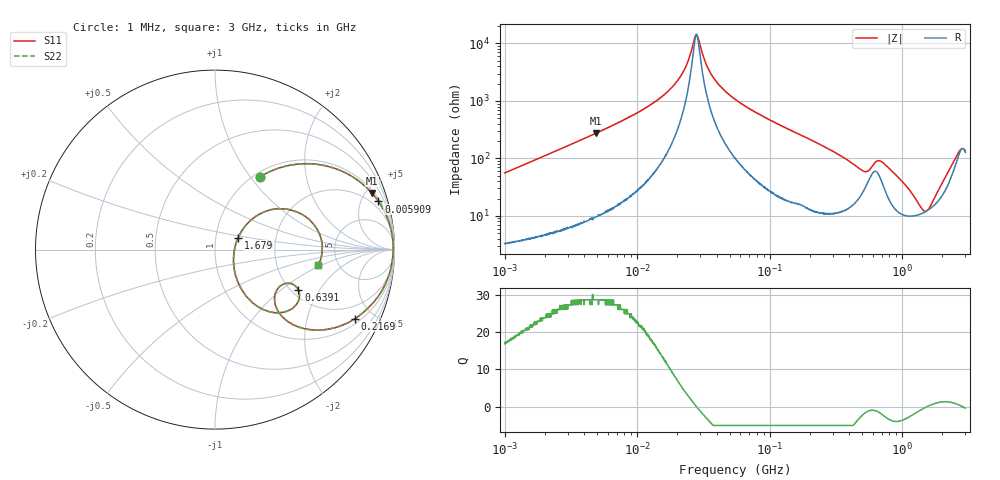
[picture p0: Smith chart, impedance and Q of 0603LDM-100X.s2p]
!s-Parameter Generated by FASTRON Sdn. Bhd.
!FASTRON P/N : 0603LDM-100X
!Keysight Technologies: E4991B_MY54100416_A.01.15
!Date: Thu Nov 27 16:25:48 2025
!Version  :Rev00  Thu Nov 27 16:25:48 2025
!Data & Calibration Information:
!Freq  S11  S21  S12  S22
!PortZ  Port1:50+j0  Port2:50+j0
!When reading reference impedance value at option line is always used.
! Remarks : This data is being provided solely for informational purposes.
# Hz S dB R 50
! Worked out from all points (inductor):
!   1601 points, 1 MHz to 3 GHz, reference 50 ohm
!   read as one part in series: L = 8.81 uH near 1.041 MHz
!   highest Q = 28.6 at 4.861 MHz (marker M1), where L = 8.92 uH
!   self-resonance near 28.01 MHz
!   S11 on the Smith chart (normalised r, x): 1 MHz: 1.07, +1.11; 5.909 MHz: 1.24, +6.72; 216.9 MHz: 1.24, -3.93; 639.1 MHz: 2.18, -1.33; 1.679 GHz: 1.29, +0.18; 3 GHz: 3.54, -0.90
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1000000  -6.46 58.3  -1.39 -28.3  -1.39 -28.3  -6.46 58.3
1926146  -2.92 42.0  -3.48 -45.5  -3.48 -45.5  -2.92 42.0
3804036  -0.99 24.9  -7.50 -63.1  -7.50 -63.1  -0.99 24.9
4861065  -0.64 19.9  -9.36 -68.1  -9.36 -68.1  -0.64 19.9
5908623  -0.45 16.4  -11.00 -71.6  -11.00 -71.6  -0.45 16.4
1.447069e7  -0.09 5.3  -20.70 -80.9  -20.70 -80.9  -0.09 5.3
2.170294e7  -0.06 1.9  -29.30 -77.4  -29.30 -77.4  -0.06 1.9
2.801249e7  -0.06 0.0  -43.20 -1.8  -43.20 -1.8  -0.06 0.0
3.652005e7  -0.07 -2.0  -29.10 75.7  -29.10 75.7  -0.07 -2.0
5.504702e7  -0.11 -5.3  -20.60 79.3  -20.60 79.3  -0.11 -5.3
2.083556e8  -1.12 -25.2  -7.40 61.3  -7.40 61.3  -1.12 -25.2
2.168657e8  -1.21 -26.2  -7.08 60.3  -7.08 60.3  -1.21 -26.2
3.523638e8  -3.16 -39.9  -3.80 43.7  -3.80 43.7  -3.16 -39.9
4.878085e8  -6.60 -43.3  -2.69 26.0  -2.69 26.0  -6.60 -43.3
5.528145e8  -7.70 -31.4  -3.32 18.3  -3.32 18.3  -7.70 -31.4
6.391491e8  -5.75 -25.8  -4.72 22.7  -4.72 22.7  -5.75 -25.8
7.925923e8  -6.02 -44.7  -2.68 28.6  -2.68 28.6  -6.02 -44.7
1.075512e9  -10.80 -56.4  -1.17 15.9  -1.17 15.9  -10.80 -56.4
1.452135e9  -19.10 -20.6  -0.94 2.5  -0.94 2.5  -19.10 -20.6
1.67892e9  -16.70 27.3  -1.18 -4.4  -1.18 -4.4  -16.70 27.3
2.335937e9  -6.75 29.3  -3.87 -20.6  -3.87 -20.6  -6.75 29.3
3e9  -4.70 -8.3  -7.29 11.2  -7.29 11.2  -4.70 -8.3
